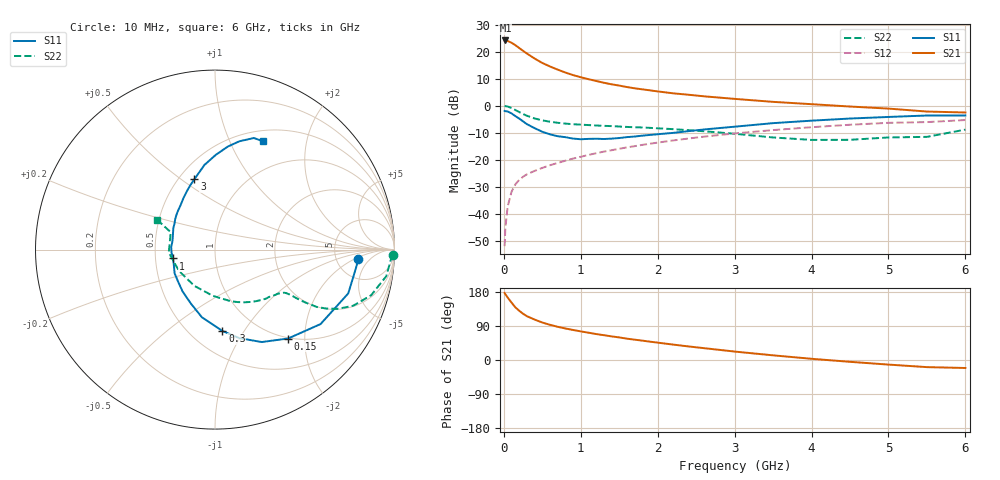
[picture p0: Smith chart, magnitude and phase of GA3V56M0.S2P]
! Infineon Technologies  Discrete & RF Semiconductors
! BF775
! Si NPN RF Bipolar Junction Transistor in SOT23
! VCE = 3.5 V  IC = 6 mA
! Common Emitter S-Parameters:  May  1996
# GHz  S  MA  R  50
!  f  S11  S21  S12  S22
! GHz  MAG  ANG  MAG  ANG  MAG  ANG  MAG  ANG
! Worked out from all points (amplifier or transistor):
!   36 points, 10 MHz to 6 GHz, reference 50 ohm
!   highest |S21| = 24.2 dB at 20 MHz (marker M1)
!   |S21| within 3 dB of that: start of sweep to 209.5 MHz
!   unconditionally stable (mu >= 1): 738.9 MHz to 3.384 GHz
!   at 250 MHz: K = 0.53, MSG = 23.3 dB, |S12| = -26.3 dB
!   at 1.4 GHz: K = 1.12, MAG = 10.1 dB, |S12| = -16.5 dB
!   at 6 GHz: K = 0.95, MSG = 1.4 dB, |S12| = -5.3 dB
!   S11 on the Smith chart (normalised r, x): 10 MHz: 8.27, -2.43; 150 MHz: 0.99, -1.66; 300 MHz: 0.70, -0.81; 1 GHz: 0.62, -0.06; 3 GHz: 0.60, +0.56; 6 GHz: 0.63, +1.34
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0.01  0.7999 -3.8  16.14 176.9  0.0025 88.2  0.9907 -1.7
0.02  0.792 -7.5  16.17 173.5  0.0055 84.9  0.9801 -3.6
0.05  0.7815 -18.2  15.78 164.8  0.0136 79.6  0.9659 -8.8
0.1  0.7198 -35.2  14.64 151.5  0.0255 72.6  0.9064 -16.3
0.15  0.6411 -50.6  13.22 138.9  0.0349 65.9  0.831 -22.1
0.2  0.5774 -63.1  11.71 129.9  0.0423 62.6  0.7629 -25.6
0.25  0.512 -74.6  10.38 122.0  0.0483 59.8  0.7022 -27.9
0.3  0.4552 -84.8  9.255 115.6  0.0536 58.5  0.6511 -29.4
0.4  0.3838 -101.0  7.479 106.7  0.062 57.7  0.5799 -30.4
0.5  0.3289 -114.2  6.187 98.9  0.0704 57.6  0.5351 -30.8
0.6  0.2948 -127.8  5.327 92.9  0.079 58.1  0.505 -30.9
0.7  0.2722 -139.1  4.656 87.6  0.087 58.8  0.4827 -31.1
0.8  0.261 -149.6  4.113 83.2  0.0957 59.1  0.4662 -31.4
1  0.239 -168.1  3.366 75.5  0.1132 59.5  0.4458 -32.8
1.1  0.2428 -176.1  3.1 72.1  0.1224 59.5  0.4376 -33.8
1.6  0.2619 152.3  2.217 56.3  0.169 57.9  0.4043 -40.1
2.2  0.3137 127.6  1.697 40.7  0.227 53.6  0.3678 -51.3
3  0.4083 106.4  1.338 22.3  0.3062 45.4  0.3018 -72.7
3.5  0.4754 97.1  1.178 12.3  0.3533 39.4  0.258 -92.6
4.5  0.5785 82.9  0.965 -4.8  0.444 26.4  0.2334 -149.4
5.5  0.6584 70.8  0.779 -18.8  0.4969 11.5  0.2648 158.6
6  0.6603 66.0  0.749 -21.1  0.5428 7.4  0.3603 152.8
